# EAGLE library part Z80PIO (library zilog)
Z80 FAMILY DEVICE
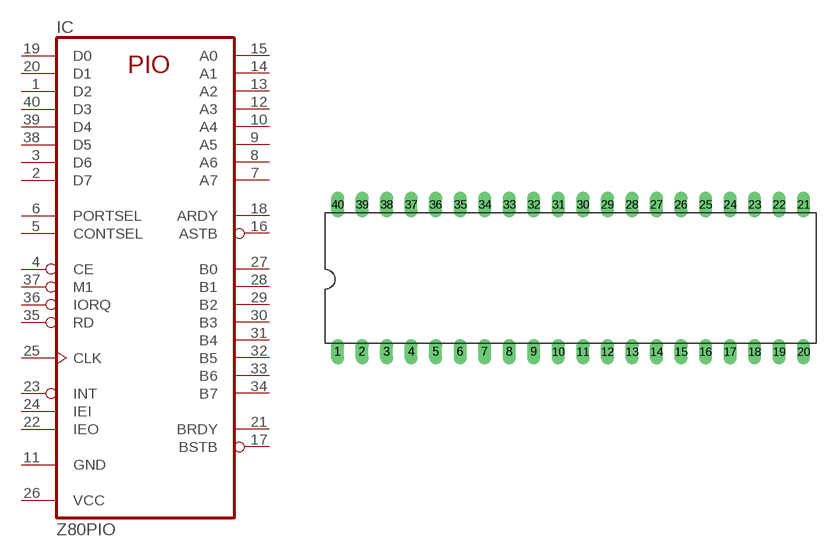
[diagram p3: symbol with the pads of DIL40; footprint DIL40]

Designator prefix IC

## Z80PIO  [DIL40]
1  D2
2  D7
3  D6
4  CE  in
5  CONTSEL  in
6  PORTSEL  in
7  A7
8  A6
9  A5
10  A4
11  GND  pwr
12  A3
13  A2
14  A1
15  A0
16  ASTB  in
17  BSTB  in
18  ARDY  out
19  D0
20  D1
21  BRDY  out
22  IEO  out
23  INT  out
24  IEI  in
25  CLK  in
26  VCC  pwr
27  B0
28  B1
29  B2
30  B3
31  B4
32  B5
33  B6
34  B7
35  RD  in
36  IORQ  in
37  M1  in
38  D5
39  D4
40  D3

## Footprint DIL40 (pad centres in mm)
Dual In Line Package
drill 0.813 long: 1 -24.13,-7.62; 2 -21.59,-7.62; 3 -19.05,-7.62; 4 -16.51,-7.62; 5 -13.97,-7.62; 6 -11.43,-7.62; 7 -8.89,-7.62; 8 -6.35,-7.62; 9 -3.81,-7.62; 10 -1.27,-7.62; 11 1.27,-7.62; 12 3.81,-7.62; 13 6.35,-7.62; 14 8.89,-7.62; 15 11.43,-7.62; 16 13.97,-7.62; 17 16.51,-7.62; 18 19.05,-7.62; 19 21.59,-7.62; 20 24.13,-7.62; 21 24.13,7.62; 22 21.59,7.62; 23 19.05,7.62; 24 16.51,7.62; 25 13.97,7.62; 26 11.43,7.62; 27 8.89,7.62; 28 6.35,7.62; 29 3.81,7.62; 30 1.27,7.62; 31 -1.27,7.62; 32 -3.81,7.62; 33 -6.35,7.62; 34 -8.89,7.62; 35 -11.43,7.62; 36 -13.97,7.62; 37 -16.51,7.62; 38 -19.05,7.62; 39 -21.59,7.62; 40 -24.13,7.62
